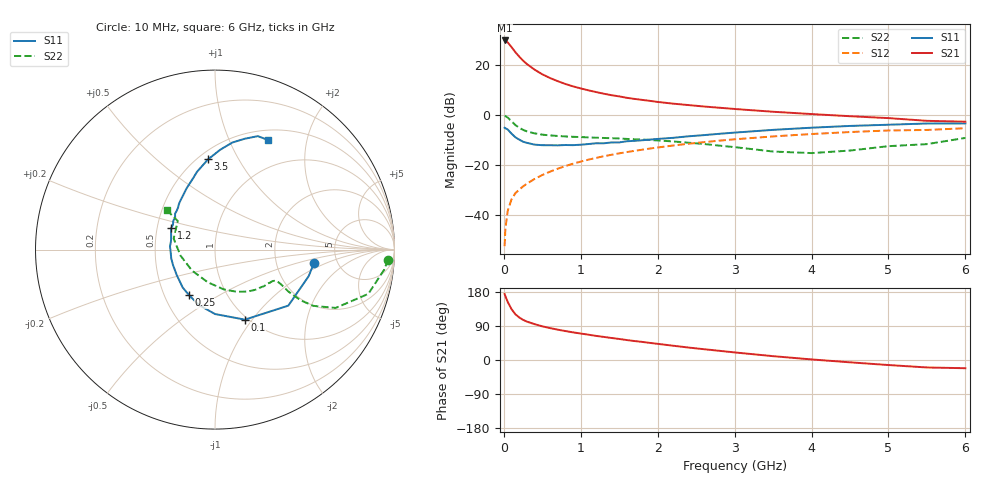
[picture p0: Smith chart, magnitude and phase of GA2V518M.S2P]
! Infineon Technologies  Discrete & RF Semiconductors
! BF775
! Si NPN RF Bipolar Junction Transistor in SOT23
! VCE = 2.5 V  IC = 18 mA
! Common Emitter S-Parameters:  May  1996
# GHz  S  MA  R  50
!  f  S11  S21  S12  S22
! GHz  MAG  ANG  MAG  ANG  MAG  ANG  MAG  ANG
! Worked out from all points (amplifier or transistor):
!   36 points, 10 MHz to 6 GHz, reference 50 ohm
!   highest |S21| = 29.8 dB at 10 MHz (marker M1)
!   |S21| within 3 dB of that: start of sweep to 108.5 MHz
!   unconditionally stable (mu >= 1): 388.8 MHz to 3.395 GHz
!   at 250 MHz: K = 0.86, MSG = 25.1 dB, |S12| = -28.5 dB
!   at 1.4 GHz: K = 1.12, MAG = 9.8 dB, |S12| = -15.9 dB
!   at 6 GHz: K = 0.97, MSG = 1.3 dB, |S12| = -5.3 dB
!   S11 on the Smith chart (normalised r, x): 10 MHz: 3.32, -0.74; 100 MHz: 0.97, -0.92; 250 MHz: 0.67, -0.37; 1.2 GHz: 0.59, +0.15; 3.5 GHz: 0.56, +0.76; 6 GHz: 0.62, +1.40
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0.01  0.5556 -8.0  30.77 174.2  0.0024 85.1  0.9658 -3.3
0.02  0.5424 -15.9  30.37 168.5  0.0053 82.6  0.949 -6.8
0.05  0.5141 -37.4  28.15 153.4  0.0121 75.8  0.8892 -16.1
0.1  0.4242 -66.9  22.67 134.1  0.0207 69.1  0.7467 -25.8
0.15  0.3591 -89.9  17.95 120.7  0.0275 64.8  0.6305 -29.8
0.2  0.3221 -106.0  14.64 112.3  0.0322 64.2  0.5558 -30.6
0.25  0.2924 -119.4  12.17 105.9  0.0375 65.3  0.5045 -30.2
0.3  0.2776 -130.4  10.39 101.3  0.0425 66.4  0.4704 -29.7
0.4  0.2559 -146.6  8.037 94.6  0.0528 67.8  0.4292 -28.2
0.5  0.2492 -159.6  6.49 88.8  0.0633 68.6  0.4045 -27.4
0.6  0.2488 -168.2  5.472 84.3  0.0738 68.9  0.3909 -27.1
0.7  0.2474 -176.8  4.737 80.1  0.0845 69.1  0.3812 -27.4
0.8  0.2514 175.9  4.16 76.4  0.0955 68.4  0.3728 -27.8
0.9  0.2497 169.2  3.728 72.9  0.1065 68.0  0.3664 -28.6
1.1  0.2629 158.7  3.106 66.8  0.1282 66.7  0.3569 -31.2
1.2  0.2722 153.9  2.869 63.6  0.1391 66.0  0.3516 -32.3
1.6  0.2989 138.1  2.202 52.6  0.1818 61.9  0.3324 -38.9
2.2  0.3497 120.7  1.683 37.7  0.2456 54.9  0.2964 -51.9
3.5  0.5043 94.4  1.16 10.1  0.3731 37.8  0.1862 -102.5
4.5  0.6043 80.8  0.945 -6.1  0.4565 24.1  0.1948 -169.9
5.5  0.6757 69.3  0.764 -19.7  0.5024 9.4  0.2616 142.4
6  0.6783 64.2  0.735 -21.7  0.5441 5.2  0.3484 140.7
